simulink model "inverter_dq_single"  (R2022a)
settings: Solver=VariableStepAuto  StartTime=0.0  StopTime=T_sim  RelTol=1e-3
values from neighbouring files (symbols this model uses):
  I_step = 1    [inverter_control_params_FR.m]
  L = Lg+Lf    (= 0.00063)    [inverter_control_params_FR.m]
  R = Rf+Rg    (= 1)    [inverter_control_params_FR.m]
  T_step = 1e-4 * 1/grid_freq0    (= 2e-06)    [inverter_control_params_FR.m]
  Vgpk = 21.5    [inverter_control_params_FR.m]

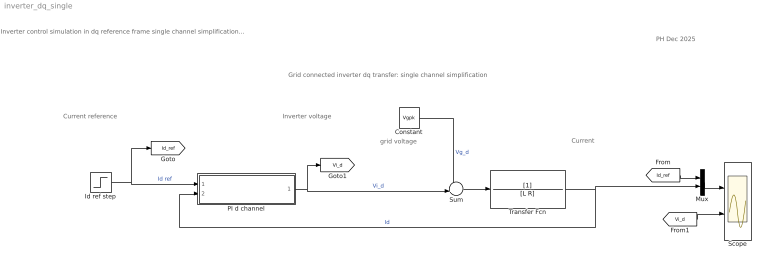
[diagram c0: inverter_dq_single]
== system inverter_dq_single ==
  note: Current reference
  note: Grid connected inverter dq transfer: single channel simplification
  note: PH Dec 2025
  note: Inverter control simulation in dq reference frame single channel simplification (here "d" represent d or q)
  note: grid voltage
  note: Inverter voltage
  note: Current
  Constant : Constant  Commented=on  Value=Vgpk
  Id ref step : Step  Time=T_step  After=I_step  SampleTime=0
  Mux : Mux  Inputs=2
  PI d channel : Subsystem  ReferencedSubsystem=pi_current
  Scope : Scope  NumInputPorts=2
  Sum : Sum  Inputs=-+|
  Transfer Fcn : TransferFcn  Denominator=[L R]
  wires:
  PI d channel/1 -> Sum/2, [Vi_d]  "Vi_d"
  Transfer Fcn/1 -> Mux/2, PI d channel/2  "Id"
  Constant/1 -> Sum/1  "Vg_d"
  Id ref step/1 -> [Id_ref], PI d channel/1  "Id ref"
  [Id_ref] -> Mux/1
  Mux/1 -> Scope/1
  [Vi_d] -> Scope/2
  Sum/1 -> Transfer Fcn/1
